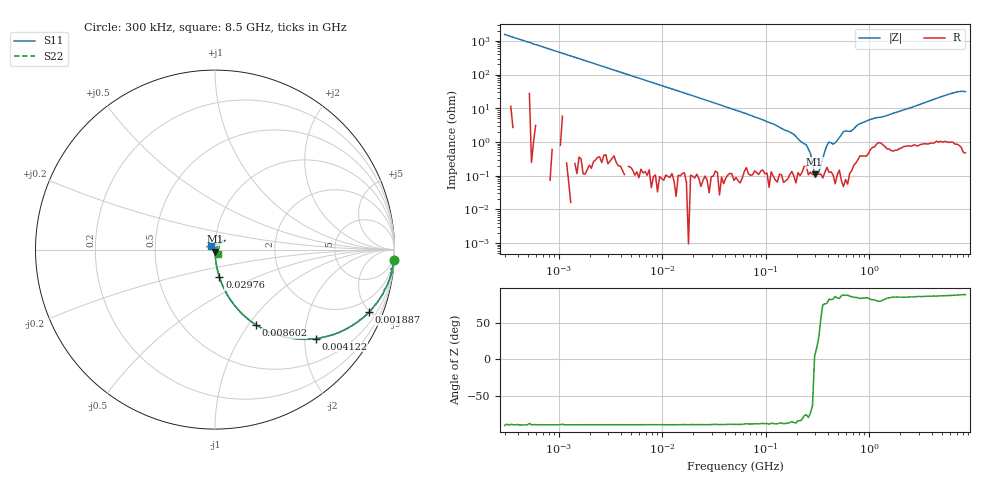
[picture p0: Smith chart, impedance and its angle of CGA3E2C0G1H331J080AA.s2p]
! S-parameter Generated by TDK Corporation
! Copyright(C) 2015 TDK Corporation.
! All Rights Reserved.
! TDK P/N: CGA3E2C0G1H331J080AA (Multilayer Ceramic Chip Capacitors)
! Property: C=330pF
! Size(LxWxT): 1.6x0.8x0.8mm, 0.063x0.031x0.031inches
! Model Type: s2p (Touchstone File Format Version 1.0)
! Frequency: DC=Yes Start=0.3MHz Stop=8500MHz 225points Log-sweep
! Note:
! Model Generated on Jun. 23, 2015
! Hash(MD5):
! Port Assignments:
!  1 ---| |--- 2
! Applicable Conditions:
!  Temperature = 25 degC
!  DC Bias Voltage = 0 V
!  Small Signal Operation
! Terms and conditions regarding TDK Simulation Models
! (1)This simulation model is being provided solely for informational purposes. Please refer to the specifications of the products in terms of detailed characteristics of such products.
! (2)In no event shall TDK Corporation of any of its subsidiaries be liable for any loss or damage arising, directly or indirectly,
!  From any information contained in this simulation model, including, but not limited to loss or damages arising from any inaccuracies, omissions or errors in connection with such information.
! (3)Any and all copyrights on this simulation model are owned by TDK Corporation.
!  Duplication or redistribution of this simulation model without prior written permission from TDK Corporation is prohibited.
! (4)This simulation model is subject to any modification or change without any prior notice.
! (5)Neither TDK Corporation nor any of its subsidiaries shall make any warranty, express or implied,
!  Including but not limited to the correctness, implied warranties of merchantability and fitness for a particular purpose with respect to this simulation models.
! (6)The use of this simulation model shall be deemed to have consented to the terms and conditions hereof.
# MHz S MA R 50
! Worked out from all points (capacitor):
!   224 points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, 300 kHz to 8.5 GHz, reference 50 ohm
!   read as one part in series: C = 341 pF near 314.1 kHz
!   lowest |Z| = 110 mohm at 296.4 MHz (marker M1)
!   series resonance near 296 MHz, so ESL is about 850 pH
!   S11 on the Smith chart (normalised r, x): 300 kHz: 1, -34; 1.887 MHz: 1.00, -4.95; 4.122 MHz: 1.00, -2.26; 8.602 MHz: 1.00, -1.08; 29.76 MHz: 1.00, -0.31; 8.5 GHz: 0.96, +0.04
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0.3  0.9979 -3.4  0.06446 87.6  0.06446 85.7  0.9979 -3.4
1.72111  0.938 -20.2  0.3462 69.8  0.3459 69.7  0.9377 -20.2
1.88686  0.9271 -22.0  0.3748 68.0  0.3748 68.0  0.9271 -22.0
4.122422  0.7484 -41.5  0.6623 48.5  0.6621 48.5  0.749 -41.5
8.602008  0.4762 -61.5  0.8785 28.4  0.8785 28.4  0.4767 -61.5
9.430415  0.4432 -63.7  0.8959 26.2  0.8958 26.3  0.4432 -63.6
29.76236  0.1545 -81.0  0.9873 8.7  0.987 8.8  0.1545 -80.9
51.67171  0.08913 -84.4  0.9947 4.9  0.9954 4.9  0.08887 -84.6
283.1228  0.01193 -85.7  0.9984 -0.4  0.9983 -0.4  0.01064 -89.2
296.4424  0.01108 -86.5  0.9988 -0.6  0.9978 -0.6  0.009614 -88.3
448.3627  0.004812 -75.7  0.9978 -1.2  0.9982 -1.2  0.002713 -116.1
514.6664  0.001527 -68.7  0.9978 -1.6  0.9963 -1.6  0.001242 -121.6
590.7752  0.001112 5.0  0.9981 -2.4  0.9985 -2.4  0.002084 131.9
618.5683  0.001837 54.0  1 -2.3  0.9978 -2.3  0.001464 129.0
710.042  0.004207 50.4  0.9966 -2.6  0.9967 -2.6  0.003025 107.8
979.5854  0.008544 73.5  0.9948 -4.6  0.9944 -4.6  0.008626 48.0
1177.346  0.01038 51.8  0.9914 -5.5  0.9895 -5.4  0.01252 32.8
1551.304  0.006436 48.8  0.9925 -7.0  0.9925 -7.0  0.008193 33.8
2572.272  0.01123 49.6  0.9914 -11.7  0.9908 -11.7  0.01169 41.0
6450.987  0.0754 42.3  0.9837 -29.6  0.9848 -29.7  0.07281 66.9
7404.957  0.06984 42.2  0.9855 -33.9  0.984 -34.0  0.06615 62.5
8500  0.02869 138.5  0.9881 -38.7  0.9874 -38.6  0.03037 -53.6
